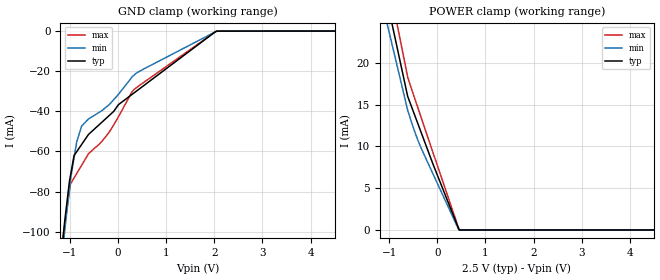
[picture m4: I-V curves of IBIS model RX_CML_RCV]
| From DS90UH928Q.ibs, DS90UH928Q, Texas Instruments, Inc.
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|   Model
[Model]   RX_CML_RCV
Model_type   Input
Vinl = 2.2
Vinh = 2.4
|   typ   min   max
C_comp   0.9027pF   0.8382pF   0.9749pF
[Voltage Range]   3.3   3.0   3.6
[Temperature Range]   25   105   -40
[Power Clamp Reference]   2.5   2.4999   2.5001 | the driver power is regulated at 2.5V
[GND Clamp Reference]   0   0   0
[GND Clamp]
|   Voltage   I(typ)   I(min)   I(max)
-3.3V     -721.1mA   -720.6mA   -785.3mA
-1.15V    -104.9mA   -109.5mA   -102.8mA
-1.128V   -98.63mA   -103.6mA   -99.07mA
-1.113V   -95.05mA   -99.83mA   -96.51mA
-992.5mV  -72.17mA   -74.75mA   -76.24mA
-917.6mV  -62.03mA   -63.36mA   -73.22mA
-857.5mV  -59.92mA   -54.86mA   -70.8mA
-760mV    -56.51mA   -47.35mA   -66.87mA
-182.5mV  -41.99mA   -36.56mA   -50.18mA
320mV     -30.99mA   -22.15mA   -29.37mA
2.045V    -25.61uA   -83.27uA   -98.91uA
6.6V      0A         0A         0A
[POWER Clamp]
|   Voltage   I(typ)   I(min)   I(max)
-3.3V     432.7mA    396.3mA    468mA
-1.367V   35.99mA    32.53mA    39.85mA
-617.6mV  15.99mA    14.34mA    18.3mA
-467.5mV  13.68mA    11.71mA    15.69mA
-355mV    11.95mA    10.05mA    13.76mA
-92.62mV  7.908mA    6.735mA    9.295mA
447.5mV   85.6uA     11.45uA    142.8uA
455mV     42.44uA    5.72uA     15.8uA
470mV     0A         0A         0A
6.6V      0A         0A         0A
